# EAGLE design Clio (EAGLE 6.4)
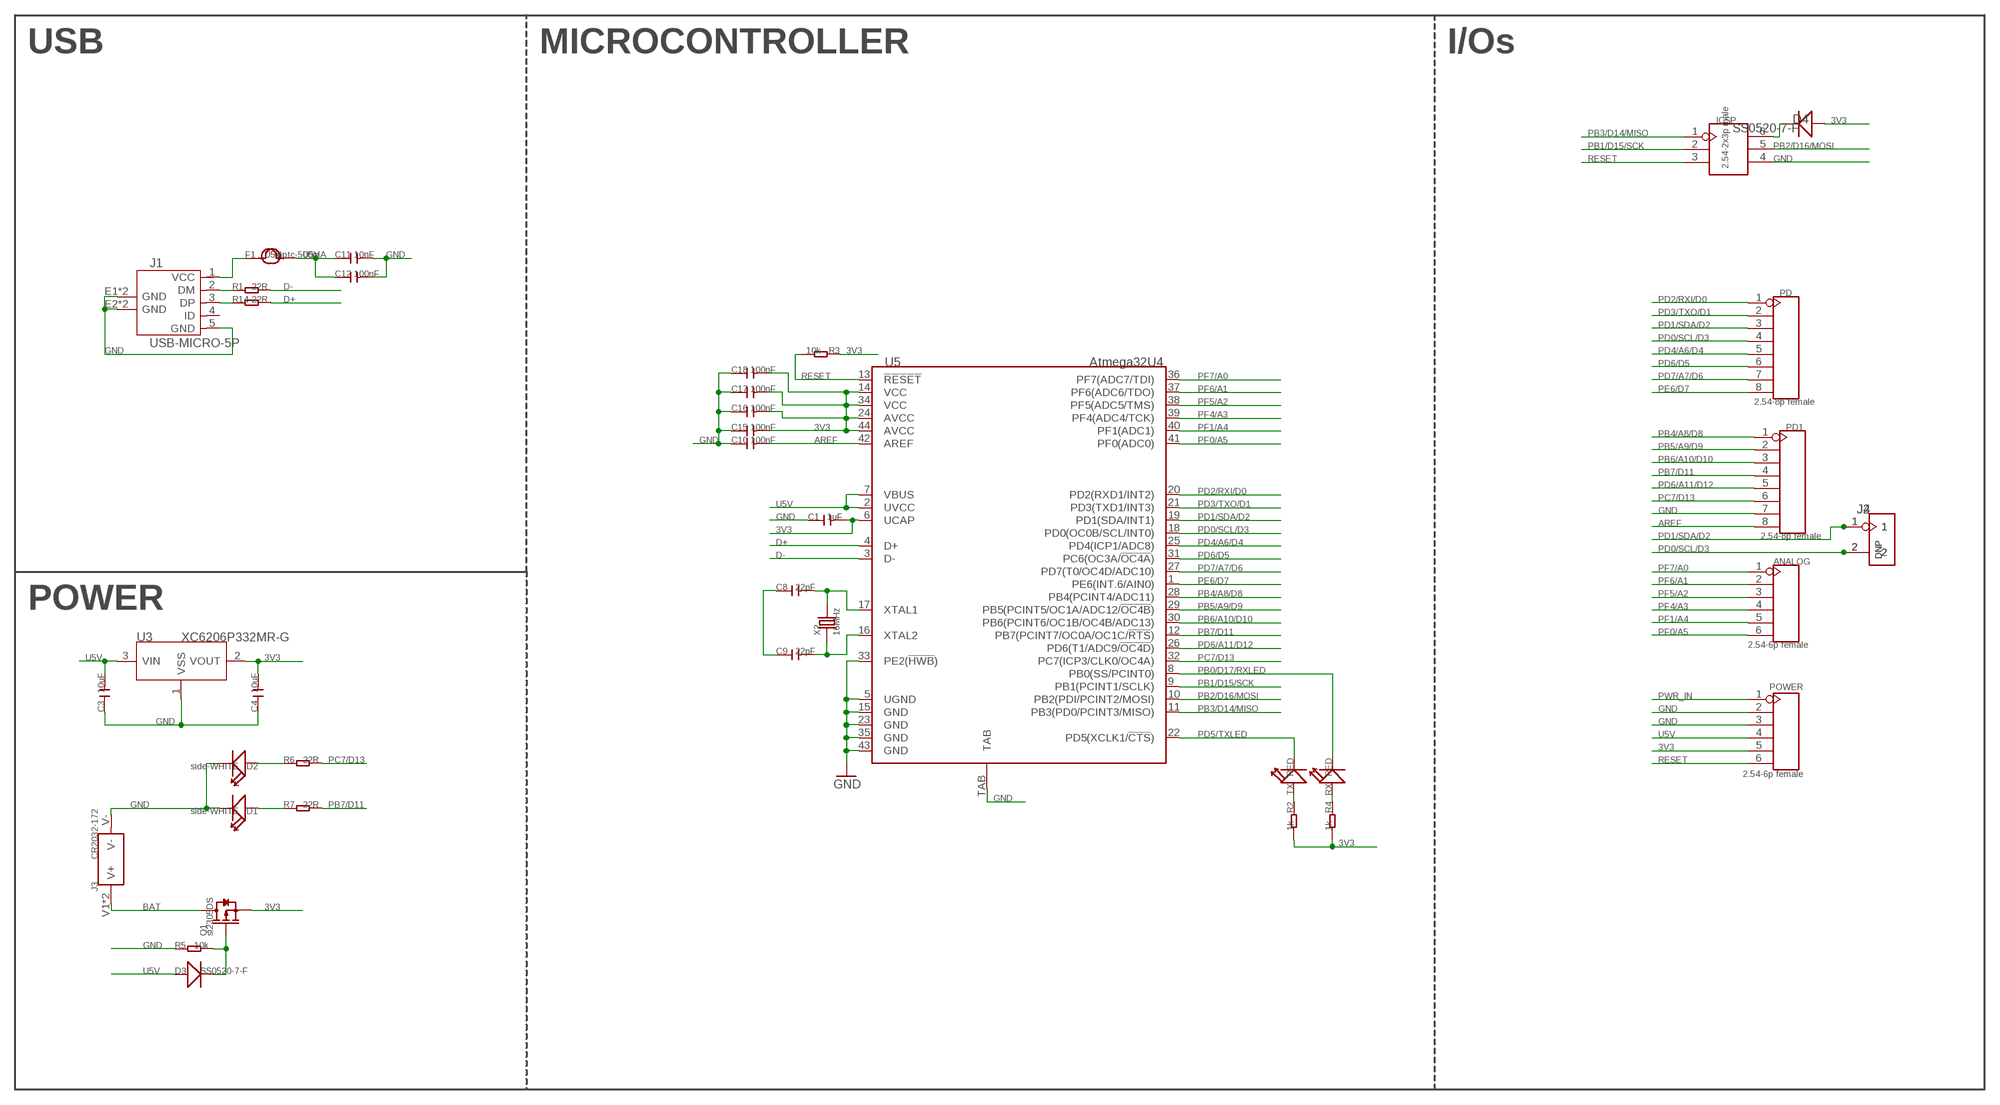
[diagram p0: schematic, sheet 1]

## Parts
ANALOG  2.54-6p female  HEADER-6P-65/35MIL  [6P-2.54-65/35MIL]
C1  1uF  C-0805  [C0805]
C3  10uF  C-0805  [C0805]
C4  10uF  C-0805  [C0805]
C8  22pF  C-0603  [C0603]
C9  22pF  C-0603  [C0603]
C10  100nF  C-0603  [C0603]
C11  10nF  C-0603  [C0603]
C12  100nF  C-0603  [C0603]
C15  100nF  C-0603  [C0603]
C16  100nF  C-0603  [C0603]
C17  100nF  C-0603  [C0603]
C18  100nF  C-0603  [C0603]
D1  side-WHITE  LED'RIGHT'  [LED-SIDE-VIEW-0603-RIGHT]
D2  side-WHITE  LED'RIGHT'  [LED-SIDE-VIEW-0603-RIGHT]
D3  SS0520-7-F  D'1206'  [SOD123]
D4  SS0520-7-F  D'1206'  [SOD123]
F1  pptc-500mA  FUSE'1206'  [F1206]
ICSP  2.54-2x3p male  HEADER-2X3P-2.54  [2X3P-2.54]
J1  USB-MICRO-5P  [MICRO-USB-5P]
J2  DNP  HEADER-2P-65/35MIL  [2P-2.54-65/35MIL]
J3  CR2032-172  HOLDER-BAT-D20.32  [2032-SMD-D20.32]
J4  DNP  HEADER-2P-65/35MIL  [2P-2.54-65/35MIL]
PD  2.54-8p female  HEADER-8P-2.54  [8P-2.54]
PD1  2.54-8p female  HEADER-8P-2.54  [8P-2.54]
POWER  2.54-6p female  HEADER-6P-65/35MIL  [6P-2.54-65/35MIL]
Q1  si2305DS  MOSFET-P'SI2323CDS/SI2305DS<BR>'  [SOT23]
R1  22R  R-0603  [R0603]
R2  1k  R-0603  [R0603]
R3  10k  R-0603  [R0603]
R4  1k  R-0603  [R0603]
R5  10k  R-0603  [R0603]
R6  22R  R-0603  [R0603]
R7  22R  R-0603  [R0603]
R14  22R  R-0603  [R0603]
RX  RED  LED'0603'  [LED-0603]
TX  RED  LED'0603'  [LED-0603]
U3  XC6206P332MR-G  XC6206MR  [SOT23]
U5  Atmega32U4  ATMEGA32U4-QFN44  [QFN44]
X2  16MHz  CRYSTAL'5032'  [2P-SMD-5X3.2]

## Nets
3V3: C1.2 C4.2 C15.2 C16.2 C17.2 C18.2 D4.+ POWER.5 Q1.2(S) R2.2 R3.1 R4.2 U3.2(VOUT) U5.6(UCAP) U5.14(VCC) U5.24(AVCC) U5.34(VCC) U5.44(AVCC)
AREF: C10.2 PD1.8 U5.42(AREF)
BAT: J3.V1(V+) J3.V2(V+) Q1.3(D)
D+: R14.2 U5.4(D+)
D-: R1.2 U5.3(D-)
GND: C1.1 C3.1 C4.1 C8.1 C9.1 C10.1 C11.2 C12.2 C15.1 C16.1 C17.1 C18.1 D1.2(-) D2.2(-) ICSP.4 J1.5(GND) J1.E1(GND) J1.E2(GND) J1.P1(GND) J1.P2(GND) J3.V- PD1.7 POWER.2 POWER.3 R5.1 U3.1(VSS) U5.5(UGND) U5.15(GND) U5.23(GND) U5.33(PE2(!HWB!)) U5.35(GND) U5.43(GND) U5.TAB
N$1: C8.2 U5.17(XTAL1) X2.2
N$2: C9.2 U5.16(XTAL2) X2.1
N$3: R2.1 TX.+
N$4: D3.- Q1.1(G) R5.2
N$5: R4.1 RX.+
N$6: J1.3(DP) R14.1
N$7: D1.1(+) R7.1
N$8: J1.2(DM) R1.1
N$9: F1.1 J1.1(VCC)
N$11: D2.1(+) R6.1
N$13: D4.- ICSP.6
PB0/D17/RXLED: RX.- U5.8(PB0(SS/PCINT0))
PB1/D15/SCK: ICSP.2 U5.9(PB1(PCINT1/SCLK))
PB2/D16/MOSI: ICSP.5 U5.10(PB2(PDI/PCINT2/MOSI))
PB3/D14/MISO: ICSP.1 U5.11(PB3(PD0/PCINT3/MISO))
PB4/A8/D8: PD1.1 U5.28(PB4(PCINT4/ADC11))
PB5/A9/D9: PD1.2 U5.29(PB5(PCINT5/OC1A/ADC12/!OC4B!))
PB6/A10/D10: PD1.3 U5.30(PB6(PCINT6/OC1B/OC4B/ADC13))
PB7/D11: PD1.4 R7.2 U5.12(PB7(PCINT7/OC0A/OC1C/!RTS!))
PC7/D13: PD1.6 R6.2 U5.32(PC7(ICP3/CLK0/OC4A))
PD0/SCL/D3: J2.2 J4.2 PD.4 U5.18(PD0(OC0B/SCL/INT0))
PD1/SDA/D2: J2.1 J4.1 PD.3 U5.19(PD1(SDA/INT1))
PD2/RXI/D0: PD.1 U5.20(PD2(RXD1/INT2))
PD3/TXO/D1: PD.2 U5.21(PD3(TXD1/INT3))
PD4/A6/D4: PD.5 U5.25(PD4(ICP1/ADC8))
PD5/TXLED: TX.- U5.22(PD5(XCLK1/!CTS!))
PD6/A11/D12: PD1.5 U5.26(PD6(T1/ADC9/!OC4D!))
PD6/D5: PD.6 U5.31(PC6(OC3A/!OC4A!))
PD7/A7/D6: PD.7 U5.27(PD7(T0/OC4D/ADC10))
PE6/D7: PD.8 U5.1(PE6(INT.6/AIN0))
PF0/A5: ANALOG.6 U5.41(PF0(ADC0))
PF1/A4: ANALOG.5 U5.40(PF1(ADC1))
PF4/A3: ANALOG.4 U5.39(PF4(ADC4/TCK))
PF5/A2: ANALOG.3 U5.38(PF5(ADC5/TMS))
PF6/A1: ANALOG.2 U5.37(PF6(ADC6/TDO))
PF7/A0: ANALOG.1 U5.36(PF7(ADC7/TDI))
PWR_IN: POWER.1
RESET: ICSP.3 POWER.6 R3.2 U5.13(!RESET)
U5V [usbvcc]: C3.2 C11.1 C12.1 D3.+ F1.2 POWER.4 U3.3(VIN) U5.2(UVCC) U5.7(VBUS)
Unconnected: J1.4(ID)

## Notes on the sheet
- USB | MICROCONTROLLER | I/Os
- POWER

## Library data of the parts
ANALOG POWER = Connector:HEADER-6P
C1 C3 C4 C8-C12 C15-C18 = Discrete:C*: Ceramic Capacitors
D1 D2 RX TX = Discrete:LED*
D3 D4 = Discrete:D*
F1 = Discrete:FUSE
ICSP = Connector:HEADER-2X3P
J1 = Connector:USB-MICRO-5P
J2 J4 = Connector:HEADER-2P
J3 = Connector:HOLDER-BAT: button cell holder
PD PD1 = Connector:HEADER-8P
Q1 = Discrete:MOSFET-P
R1-R7 R14 = Discrete:R*
U3 = IC:XC6206: LOW ESR Cap.Compatible Positive Voltage Regulators
U5 = IC:ATMEGA32U4-QFN44: 8-bit Microcontroller With 16/32K Bytes of ISP Flash and USB controller
X2 = Discrete:CRYSTAL*: CRYSTAL

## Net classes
0 default: width 0.203 mm, drill 0.305 mm, clearance 0.152 mm

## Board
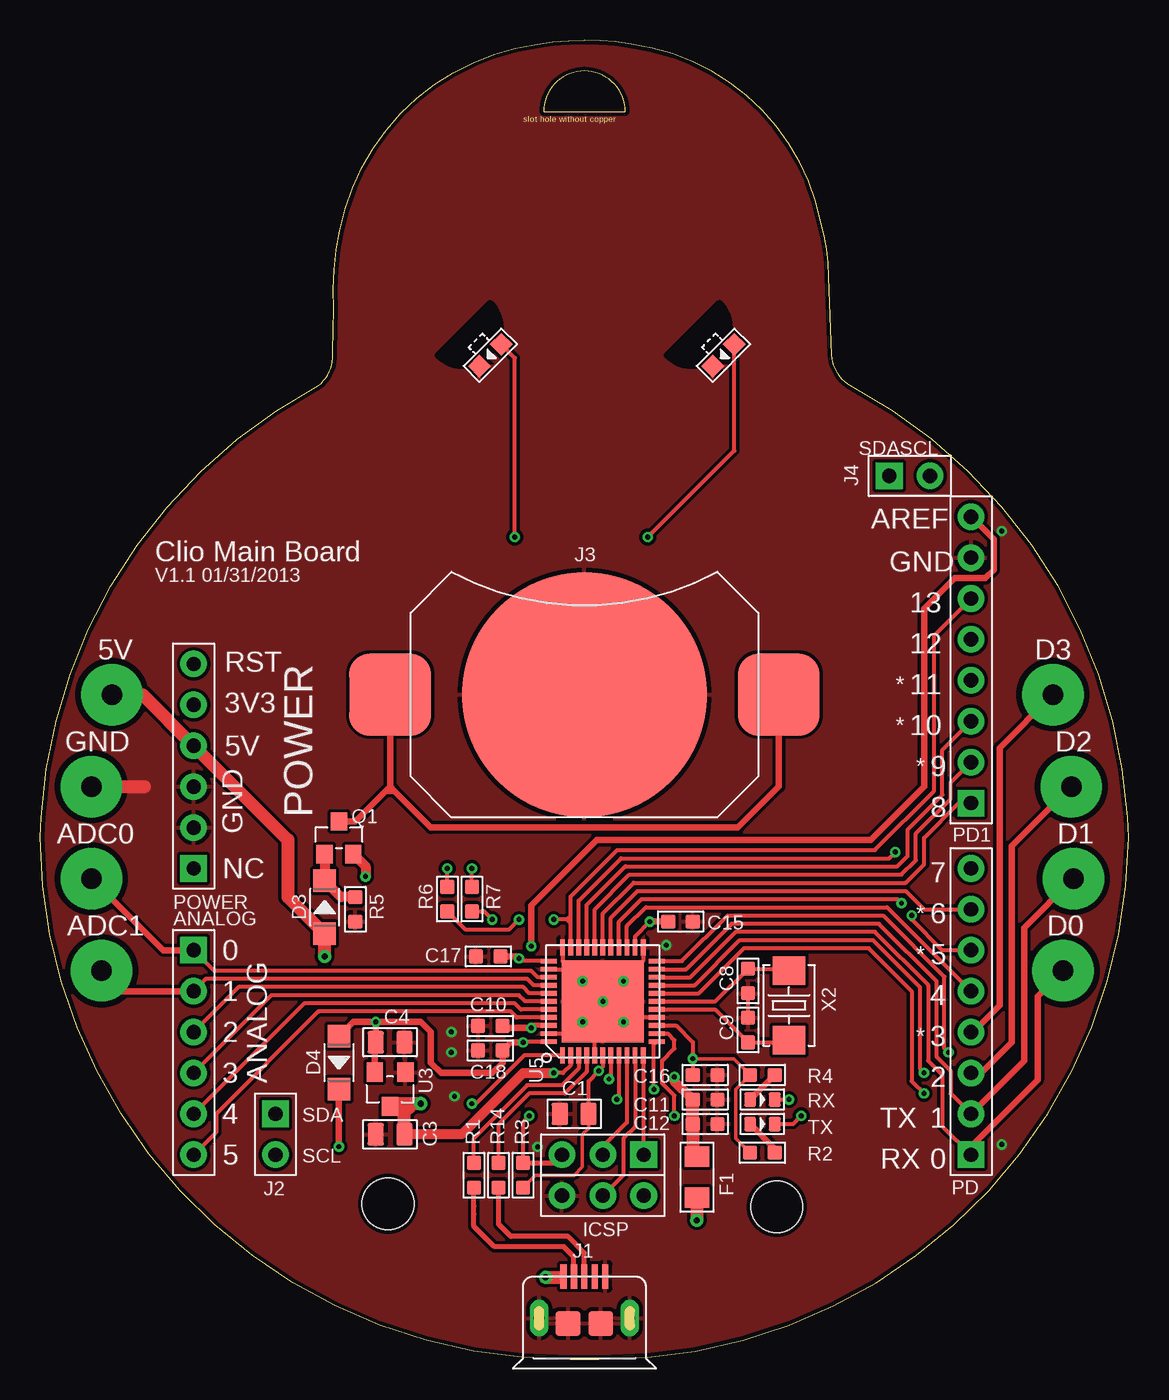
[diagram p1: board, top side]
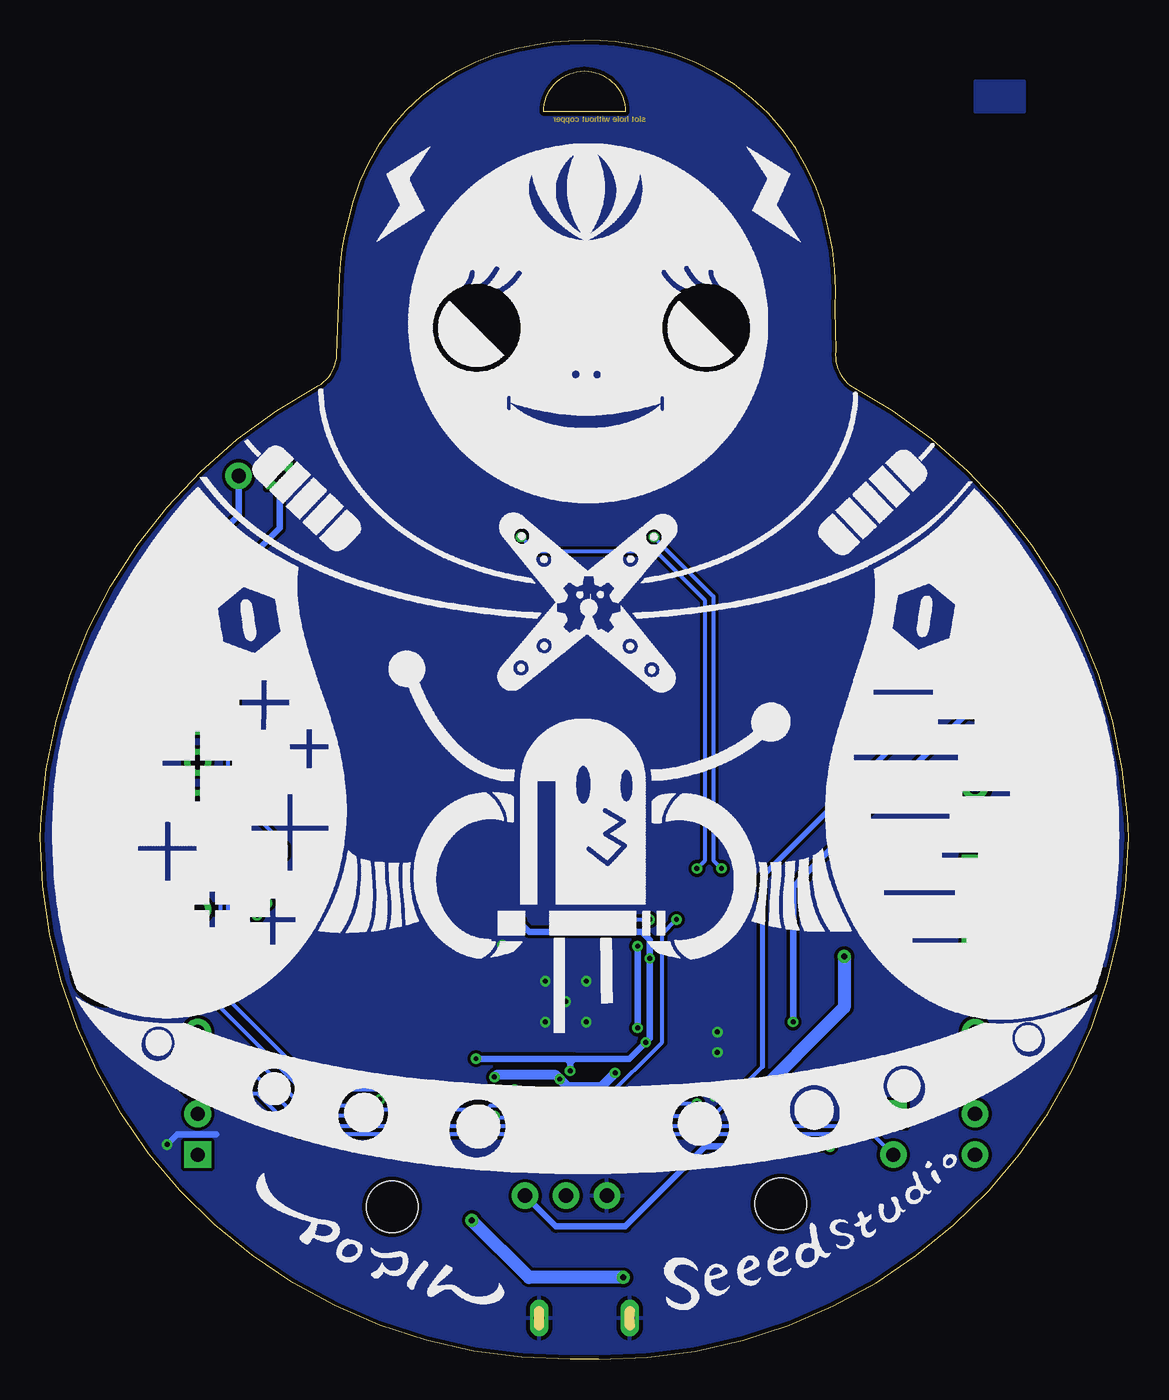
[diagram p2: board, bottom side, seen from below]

Size 67.56 x 81.92 mm. Coordinates in mm from the lower left corner, seen from the top.
Outline: 32.9,0 arc-90 0,32.39 0.06,33.66 arc-59 17.27,60.45 arc55 18.16,62.61 18.22,65.22 arc-16 18.6,70.1 arc-72 30.86,81.66 arc-11 33.78,81.92 arc-11 36.7,81.66 arc-72 48.45,70.61 arc-16 48.96,67.25 49.15,62.36 arc55 50.29,60.45 arc-59 67.5,33.66 67.56,32.39 arc-90 34.66,0 32.9,0
Outline: 31.24,77.47 36.32,77.47 arc90 33.78,80.01 arc90 31.24,77.47
Copper layers (1*16): Top 0.035mm / dielectric 1.5mm / Bottom 0.035mm
Design rules "default *": minimum track width 8mil, minimum drill 12mil, track to track 6mil, track to pad 6mil, pad to pad 6mil, via to via 6mil, smd to smd 0mil, copper to edge 10mil, drill to drill 10mil, minimum pad ring 10mil, minimum via ring 6mil, stop-mask expansion 2mil, vias tented up to drill 25mil, thermal gap 10mil
Holes 3.2 mm at 21.59,9.65 45.72,9.46
tRestrict: area 38.9,61.7 to 42.8,65.6; area 24.7,61.7 to 28.6,65.6; area 2.4,39.2 to 6.5,43.3; area -5.1,39.2 to -1,43.3; area 1.1,33.5 to 5.2,37.6; area 1.1,27.8 to 5.2,31.9; area 1.8,22.1 to 5.9,26.2; area 60.8,39.2 to 64.9,43.3; area 62,33.5 to 66.1,37.6; area 62.1,27.8 to 66.2,31.9; area 61.5,22.1 to 65.5,26.2
bRestrict: area 23.7,61.4 to 28.9,66.6; area 37.9,61.4 to 43.1,66.6; area 27.8,62.4 to 27.9,62.5; area 2.4,39.2 to 6.5,43.3; area -5.1,39.2 to -1,43.3; area 1.1,33.5 to 5.2,37.6; area 1.1,27.8 to 5.2,31.9; area 1.8,22.1 to 5.9,26.2; area 60.8,39.2 to 64.9,43.3; area 62,33.5 to 66.1,37.6; area 62.1,27.8 to 66.2,31.9; area 61.5,22.1 to 65.5,26.2
Milling: area 31.2,77.5 to 36.3,80

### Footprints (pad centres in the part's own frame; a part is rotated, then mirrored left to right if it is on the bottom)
6P-2.54-65/35MIL = drill 0.889 pad 1.651 square: 1 0,6.35 | drill 0.889 pad 1.651: 2 0,3.81; 3 0,1.27; 4 0,-1.27; 5 0,-3.81; 6 0,-6.35
C0805 = smd 1.016 x 1.397: 1 -0.889,0; 2 0.889,0
C0603 = smd 0.889 x 0.889: 1 -0.762,0; 2 0.762,0
LED-SIDE-VIEW-0603-RIGHT = smd 1 x 1: 1 0,-0.95; 2 0,0.95
SOD123 = smd 1.397 x 1.397: + -1.651,0; - 1.651,0
F1206 = smd 1.27 x 1.524: 1 -1.27,0; 2 1.27,0
2X3P-2.54 = drill 0.889 pad 1.651 square: 1 -1.27,2.54 | drill 0.889 pad 1.651: 2 -1.27,0; 3 -1.27,-2.54; 4 1.27,-2.54; 5 1.27,0; 6 1.27,2.54
MICRO-USB-5P = smd 0.38 x 1.52: 1 -1.3,0; 2 -0.65,0; 3 0,0; 4 0.65,0; 5 1.3,0 | smd 1.524 x 1.524: E1 -1.016,-2.921; E2 1.016,-2.921 | drill 0.635 pad 1.143 long: P1 -2.819,-2.591; P2 2.819,-2.591
2P-2.54-65/35MIL = drill 0.889 pad 1.651 square: 1 0,1.27 | drill 0.889 pad 1.651: 2 0,-1.27
2032-SMD-D20.32 = smd 5.08 x 5.08: V1 -12.065,0; V2 12.065,0 | smd 15.24 x 15.24: V- 0,0
8P-2.54 = drill 0.889 pad 1.651 square: 1 0,8.89 | drill 0.889 pad 1.651: 2 0,6.35; 3 0,3.81; 4 0,1.27; 5 0,-1.27; 6 0,-3.81; 7 0,-6.35; 8 0,-8.89
SOT23 = smd 1.016 x 1.143: 1 -0.889,-1.016; 2 0.889,-1.016; 3 0,1.016
R0603 = smd 0.889 x 0.889: 1 -0.762,0; 2 0.762,0
LED-0603 = smd 0.762 x 0.889: + -0.762,0; - 0.762,0
SOT23' = smd 1.016 x 1.2: 1 -0.95,-1.06; 2 0.95,-1.06; 3 0,1.06
QFN44 = smd 1 x 0.3: 1 -3.35,2.5; 2 -3.35,2; 3 -3.35,1.5; 4 -3.35,1; 5 -3.35,0.5; 6 -3.35,0; 7 -3.35,-0.5; 8 -3.35,-1; 9 -3.35,-1.5; 10 -3.35,-2; 11 -3.35,-2.5; 23 3.35,-2.5; 24 3.35,-2; 25 3.35,-1.5; 26 3.35,-1; 27 3.35,-0.5; 28 3.35,0; 29 3.35,0.5; 30 3.35,1; 31 3.35,1.5; 32 3.35,2; 33 3.35,2.5 | smd 0.3 x 1: 12 -2.5,-3.35; 13 -2,-3.35; 14 -1.5,-3.35; 15 -1,-3.35; 16 -0.5,-3.35; 17 0,-3.35; 18 0.5,-3.35; 19 1,-3.35; 20 1.5,-3.35; 21 2,-3.35; 22 2.5,-3.35; 34 2.5,3.35; 35 2,3.35; 36 1.5,3.35; 37 1,3.35; 38 0.5,3.35; 39 0,3.35; 40 -0.5,3.35; 41 -1,3.35; 42 -1.5,3.35; 43 -2,3.35; 44 -2.5,3.35 | smd 5.08 x 5.08: TAB 0,0
2P-SMD-5X3.2 = smd 1.778 x 2.032: 1 -2.159,0; 2 2.159,0

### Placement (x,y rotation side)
ANALOG  9.52,19.05 0 top
C1  33.15,15.24 0 top
C3  21.72,13.97 0 top
C4  21.72,19.68 180 top
C8  43.94,23.5 90 top
C9  43.94,20.45 270 top
C10  27.94,20.7 0 top
C11  41.27,16.13 0 top
C12  41.27,14.61 0 top
C15  39.75,27.18 180 top
C16  41.27,17.65 180 top
C17  27.81,25.02 0 top
C18  27.94,19.18 0 top
D1  42.42,62.36 135 top
D2  27.94,62.36 135 top
D3  17.65,28.07 90 top
D4  18.54,18.41 270 top
F1  40.77,11.3 90 top
ICSP  34.92,11.43 270 top
J1  33.78,5.14 0 top
J2  14.6,13.97 0 top
J3  33.78,41.27 180 top
J4  53.97,54.86 90 top
PD  57.78,21.59 180 top
PD1  57.78,43.43 180 top
POWER  9.52,36.83 180 top
Q1  18.54,32.38 0 top
R1  26.92,11.43 90 top
R2  44.83,12.83 180 top
R3  29.97,11.43 90 top
R4  44.83,17.65 180 top
R5  19.56,27.94 90 top
R6  25.27,28.57 270 top
R7  26.8,28.57 270 top
R14  28.45,11.43 90 top
RX  44.83,16.13 0 top
TX  44.83,14.61 0 top
U3  XC6206P332MR-G  [SOT23']  21.72,16.76 180 top
U5  34.92,22.23 90 top
U$1  [FEMALE_BACK]  33.78,0 0 bottom
X2  46.48,21.97 90 top

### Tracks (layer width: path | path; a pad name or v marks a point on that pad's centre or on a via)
3V3  (via drill 0.3 pad 0.64)
  Top 0.203: R2.2 43.18,13.72 43.18,16.76 R4.2 43.05,18.67 v40.51,18.67 | R3.1 30.73,11.43 33.15,11.43 33.65,11.94 33.65,13.97 34.04,14.35 C1.2
  Top 0.254: U5.14 39.48,20.73 40.51,19.69 v40.51,18.67 C16.2 | U5.44 30.01,19.73 v29.97,19.68 | U5.34 29.88,24.73 v29.72,24.89 | U5.24 36.92,26.26 v37.85,27.18 | U5.6 34.92,18.16 v34.67,17.91 34.04,17.27 C1.2
  Top 0.406: v20.83,20.95 C4.2 20.77,19.62 U3.2 | v20.83,20.95 23.62,20.95 24.26,20.32 24.26,18.41 24.89,17.78 28.07,17.78 28.7,18.41 C18.2 29.21,19.68 v29.97,19.68 | C17.2 29.59,25.02 v29.72,24.89 | C15.2 v37.85,27.18 | v20.83,20.95 19.43,20.95 D4.+
  Top 0.61: Q1.2 20.19,30.61 v20.19,29.97
  Bottom 0.406: v20.83,20.95 20.83,29.34 v20.19,29.97 POWER.5 | v37.85,27.18 37.21,26.54 30.23,26.54 29.72,26.04 v29.72,24.89 29.72,19.94 v29.97,19.68 30.99,18.67 34.42,18.67 | 34.67,18.67 34.92,18.67 | 34.92,18.67 v40.51,18.67 | v34.67,17.91 34.67,18.29 34.67,18.41 | 34.67,18.41 34.67,18.67 | 34.67,18.67 34.42,18.67 | 34.67,18.41 34.42,18.67 | 34.67,18.41 34.92,18.67
AREF  (via drill 0.3 pad 0.64)
  Top 0.305: U5.42 30.63,20.73 v30.48,20.57
  Top 0.406: v30.48,25.65 30.48,28.19 34.54,32.26 51.56,32.26 54.86,35.56 54.86,46.61 56.77,48.51 58.67,48.51 59.18,49.02 59.18,50.93 PD1.8 | v30.48,20.57 28.83,20.57 C10.2
  Bottom 0.406: v30.48,25.65 v30.48,20.57
BAT
  Top 0.406: J3.V1 45.85,35.56 43.31,33.02 24.26,33.02 21.97,35.31 | 21.72,35.56 J3.V2 | 21.72,35.56 21.97,35.31 | 21.97,35.31 21.46,35.31 | 21.46,35.31 21.72,35.56 | Q1.3 19.56,33.4 21.46,35.31
D+
  Top 0.254: U5.4 33.92,17.86 32.58,16.51 30.35,16.51 28.45,14.61 R14.2
D-
  Top 0.254: U5.3 33.42,18.06 32.38,17.02 30.23,17.02 26.92,13.72 R1.2
GND  (via drill 0.3 pad 0.64, 1.27 pad 3.81)
  Top 0.254: U5.5 34.42,21.73 U5.TAB | U5.15 35.92,21.23 35.31,21.84 | 35.31,21.84 U5.TAB | U5.43 33.69,20.23 35.31,21.84 | U5.35 32.92,24.23 | 32.92,24.23 U5.TAB | U5.33 32.42,24.73 32.92,24.23 | U5.23 37.42,24.73 36.83,24.13 | C9.1 C8.1
  Top 0.813: v3.17,35.56 6.48,35.56
  Bottom 0.406: v59.69,13.34 59.05,13.97 56.64,13.97
  other vias: 38.86,25.72 25.53,20.32 25.53,19.05 25.72,16.32 34.94,22.21 33.67,23.48 36.21,23.48 36.21,20.94 33.67,20.94 59.69,51.44 30.87,13.2
  pour Bottom: 6.48,79.38 9.52,79.38 9.52,77.47 6.48,77.47
  pour Bottom (isolate 0.203, rank 6): 17.27,61.59 17.27,81.92 43.43,81.92 50.29,81.92 50.29,61.59 68.07,61.59 68.07,5.08 68.07,0 14.73,0 -0.51,0 -0.51,40.01 -0.51,61.59
  pour Top (isolate 0.203, rank 6): 17.27,61.59 17.27,81.92 43.43,81.92 50.29,81.92 50.29,61.59 68.07,61.59 68.07,5.08 68.07,0 14.73,0 -0.51,0 -0.51,40.01 -0.51,61.59
N$1
  Top 0.254: U5.17 41.91,22.23 C8.2 46.35,24.26 X2.2
N$2
  Top 0.254: U5.16 41.9,21.73 C9.2 46.35,19.68 X2.1
N$3
  Top 0.406: R2.1 45.59,13.08 TX.+
N$4
  Top 0.61: Q1.1 D3.- 18.67,28.7 R5.2
N$5
  Top 0.406: RX.+ R4.1
N$6
  Top 0.305: J1.3 33.78,6.6 32.77,7.62 29.21,7.62 28.45,8.38 R14.1
N$7  (via drill 0.3 pad 0.64)
  Top 0.254: R7.1 v26.8,30.48 | v37.72,51.05 43.09,56.42 D1.1
  Bottom 0.254: v26.8,30.48 26.29,30.99 26.29,47.12 29.34,50.16 36.83,50.16 v37.72,51.05
N$8
  Top 0.305: J1.2 33.13,6.37 32.51,6.99 28.19,6.99 26.92,8.26 26.92,9.02 26.92,9.53 R1.1
N$9  (via drill 0.38 pad 0.81)
  Top 0.254: J1.1 32.32,5.14 32.26,5.08
  Top 0.813: F1.1 v40.77,8.64 | v31.37,5.08 32.26,5.08
  Bottom 0.813: v31.37,5.08 37.21,5.08 v40.77,8.64
N$11  (via drill 0.3 pad 0.64)
  Top 0.254: R6.1 v25.27,30.48 | v29.46,51.05 29.46,62.18 D2.1
  Bottom 0.254: v29.46,51.05 25.78,47.37 25.78,30.99 v25.27,30.48
N$13  (via drill 0.3 pad 0.64)
  Top 0.406: D4.- v18.54,13.21
  Bottom 0.406: ICSP.6 35.56,8.26 31.24,8.26 26.29,13.21 v18.54,13.21
PB0/D17/RXLED  (via drill 0.3 pad 0.64)
  Top 0.254: RX.- v46.48,16.13 | U5.8 35.92,16.27 v35.8,16.14
  Bottom 0.254: v46.48,16.13 46.35,16.26 38.73,16.26 38.48,16 35.94,16 v35.8,16.14
PB1/D15/SCK
  Top 0.254: U5.9 36.42,14.71 34.92,13.21 ICSP.2
PB2/D16/MOSI
  Top 0.254: U5.10 36.92,14.45 36.19,13.72 36.19,11.43 ICSP.5
PB3/D14/MISO
  Top 0.254: U5.11 37.42,12.74 ICSP.1
PB4/A8/D8
  Top 0.254: U5.28 34.92,27.69 36.83,29.59 53.72,29.59 54.86,30.73 54.86,32.38 57.02,34.54 PD1.1
PB5/A9/D9
  Top 0.254: U5.29 34.42,27.95 36.58,30.1 53.47,30.1 54.36,30.99 54.36,32.64 56.52,34.8 56.52,35.81 PD1.2
PB6/A10/D10
  Top 0.254: U5.30 33.92,28.21 36.32,30.61 53.21,30.61 53.85,31.24 53.85,32.89 56.01,35.05 56.01,37.85 PD1.3
PB7/D11  (via drill 0.3 pad 0.64)
  Top 0.254: v38.1,16.76 38.1,19.55 U5.12 | R7.2 27.56,27.81 v28.07,27.3
  Bottom 0.254: PD1.4 55.88,40.26 55.88,22.35 50.29,16.76 v38.1,16.76 35.56,16.76 34.92,16.13 32.51,16.13 28.96,19.68 28.96,26.42 v28.07,27.3
PC7/D13  (via drill 0.3 pad 0.64)
  Top 0.254: U5.32 32.92,27.07 | 32.92,27.07 32.92,27.55 | 32.92,27.55 32.92,28.73 35.81,31.62 51.82,31.62 55.5,35.31 55.5,44.96 PD1.6 | 32.92,27.55 32.68,27.3 v31.88,27.3 32.69,27.3 32.92,27.07 | v29.72,27.3 29.08,26.67 26.42,26.67 R6.2
  Bottom 0.254: v31.88,27.3 v29.72,27.3
PD0/SCL/D3  (via drill 0.3 pad 0.64, 1.27 pad 3.81)
  Top 0.254: U5.18 40.89,22.73 43.69,25.53 51.43,25.53 54.1,22.86 54.1,17.27 v54.86,16.51
  Top 0.406: PD.4 57.91,20.32 59.56,21.97 59.56,37.97 v62.86,41.27
  Bottom 0.254: PD.4 59.15,18.96 | 59.15,18.96 | J2.2 15.87,13.97 51.56,13.97 54.1,16.51 v54.86,16.51 58.39,16.51 59.15,17.27 59.15,18.96
  Bottom 0.406: J4.2 55.24,52.43 56.62,51.05 58.93,51.05 61.09,48.9 61.09,43.05 v62.86,41.27
PD1/SDA/D2  (via drill 0.3 pad 0.64, 1.27 pad 3.81)
  Top 0.254: U5.19 40.62,23.23 43.43,26.04 51.69,26.04 54.61,23.11 54.61,18.03 v54.86,17.78
  Top 0.406: PD.3 58.42,17.78 60.32,19.68 60.32,31.88 v64.01,35.56
  Bottom 0.254: PD.3 v54.86,17.78 54.36,17.78 51.05,14.48 15.37,14.48 J2.1
  Bottom 0.406: v64.01,35.56 64.01,36.2 59.18,41.02 59.18,47.95 58.61,48.51 55.8,48.51 52.7,51.61 J4.1
PD2/RXI/D0  (via drill 1.27 pad 3.81)
  Top 0.254: U5.20 40.36,23.73 43.18,26.54 51.82,26.54 55.12,23.24 55.12,18.54 56.01,17.65 56.01,14.48 PD.1
  Top 0.406: PD.1 57.78,13.21 61.91,17.34 61.91,22.54 v63.5,24.13
PD3/TXO/D1  (via drill 1.27 pad 3.81)
  Top 0.254: U5.21 40.1,24.23 42.93,27.05 52.07,27.05 55.63,23.5 55.63,18.8 56.52,17.91 56.52,16.51 PD.2
  Top 0.406: PD.2 61.09,18.54 61.09,26.8 v64.13,29.84
PD4/A6/D4
  Top 0.254: U5.25 36.42,26.9 37.59,28.07 52.58,28.07 PD.5
PD5/TXLED  (via drill 0.3 pad 0.64)
  Top 0.254: U5.22 39.84,24.73 42.67,27.56 52.32,27.56 56.13,23.75 56.13,19.3 v56.39,19.05 | TX.- 46.74,14.61 v47.24,15.11
  Bottom 0.254: v56.39,19.05 54.61,19.05 50.67,15.11 v47.24,15.11
PD6/A11/D12  (via drill 0.3 pad 0.64)
  Top 0.254: U5.26 35.92,27.16 37.34,28.57 53.21,28.57 v53.47,28.32
  Bottom 0.254: PD1.5 55.37,42.29 55.37,34.92 52.32,31.88 52.32,31.24 53.47,30.1 v53.47,28.32
PD6/D5  (via drill 0.3 pad 0.64)
  Top 0.254: U5.31 33.42,28.47 36.07,31.11 52.7,31.11 v53.09,31.5 | PD.6 56.01,25.4 54.1,27.3 v54.1,27.56
  Bottom 0.254: v54.1,27.56 54.1,30.48 v53.09,31.5
PD7/A7/D6
  Top 0.254: U5.27 35.42,27.42 37.09,29.08 53.72,29.08 54.86,27.94 PD.7
PE6/D7  (via drill 0.3 pad 0.64)
  Top 0.254: U5.1 30.05,18.88 27.05,15.88 v26.8,15.88
  Bottom 0.254: PD.8 56.39,29.08 56.39,21.84 50.29,15.75 46.99,15.75 46.72,15.48 39.89,15.48 39.62,15.75 38.99,15.75 38.73,15.49 32.26,15.49 31.88,15.88 v26.8,15.88
PF0/A5
  Top 0.254: U5.41 29.57,21.23 29.21,21.59 17.27,21.59 10.92,15.24 10.92,14.1 ANALOG.6
PF1/A4
  Top 0.254: U5.40 29.84,21.73 29.46,22.1 16.38,22.1 ANALOG.5
PF4/A3
  Top 0.254: U5.39 30.1,22.23 29.72,22.61 14.35,22.61 ANALOG.4
PF5/A2
  Top 0.254: U5.38 30.36,22.73 29.97,23.11 12.32,23.11 ANALOG.3
PF6/A1  (via drill 1.27 pad 3.81)
  Top 0.254: U5.37 30.62,23.23 30.23,23.62 10.29,23.62 ANALOG.2
  Top 0.406: ANALOG.2 5.08,22.86 v3.81,24.13
PF7/A0  (via drill 1.27 pad 3.81)
  Top 0.254: U5.36 30.88,23.73 30.48,24.13 10.79,24.13 ANALOG.1
  Top 0.406: ANALOG.1 7.62,25.4 v3.17,29.84
RESET  (via drill 0.3 pad 0.64)
  Top 0.254: U5.13 38.96,20.23 39.37,19.81 39.37,19.3 38.61,18.54 38.61,17.14 39.37,16.38 v39.37,15.11 | R3.2 29.97,14.73 v30.35,15.11
  Top 0.305: R3.2 31.88,12.19 ICSP.3
  Bottom 0.254: 22.73,18.16 25.78,15.11 v30.35,15.11 30.48,14.99 39.24,14.99 v39.37,15.11
  Bottom 0.305: POWER.6 22.73,29.97 22.73,18.16
U5V  (via drill 0.3 pad 0.64, 0.38 pad 0.81, 1.27 pad 3.81)
  Top 0.254: U5.2 32.92,18.26 32.45,17.78 v31.88,17.78 | v35.31,17.4 35.42,17.52 U5.7
  Top 0.61: C11.1 39.37,17.27 v39.37,17.53 | C3.2 26.16,13.97 29.97,17.78 v31.88,17.78
  Top 0.813: C11.1 C12.1 40.51,12.83 F1.2 | v4.44,41.27 6.35,41.27 POWER.4 15.37,32.26 15.37,28.7 D3.+ v17.65,25.02 | 21.97,15.62 21.8,15.62 U3.3 21.89,15.88 22.35,15.88 | v23.62,15.88 22.35,15.88 | C3.2 22.61,15.37 | 22.61,15.37 22.61,15.62 22.35,15.88 | 22.61,15.37 22.99,15.75
  Bottom 0.254: 39.24,17.4 v39.37,17.53
  Bottom 0.61: v31.88,17.78 32.77,16.89 34.8,16.89 v35.31,17.4 35.56,17.65 39.24,17.65 v39.37,17.53
  Bottom 0.813: v17.65,25.02 17.65,21.84 v23.62,15.88

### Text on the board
tPlace: SDA | SCL | AREF | Clio Main Board | GND | V1.1 01/31/2013 | 13 | 12 | 5V | RST | D3 | * | 11 | 3V3 | * | 10 | GND | D2 | 5V | * | 9 | POWER | 8 | GND | ADC0 | D1 | NC | 7 | * | 6 | ADC1 | D0 | 0 | * | 5 | 1 | 4 | 2 | * | 3 | 3 | ANALOG | 2 | 4 | SDA | TX | 1 | 5 | SCL | RX | 0
Milling: slot hole without copper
